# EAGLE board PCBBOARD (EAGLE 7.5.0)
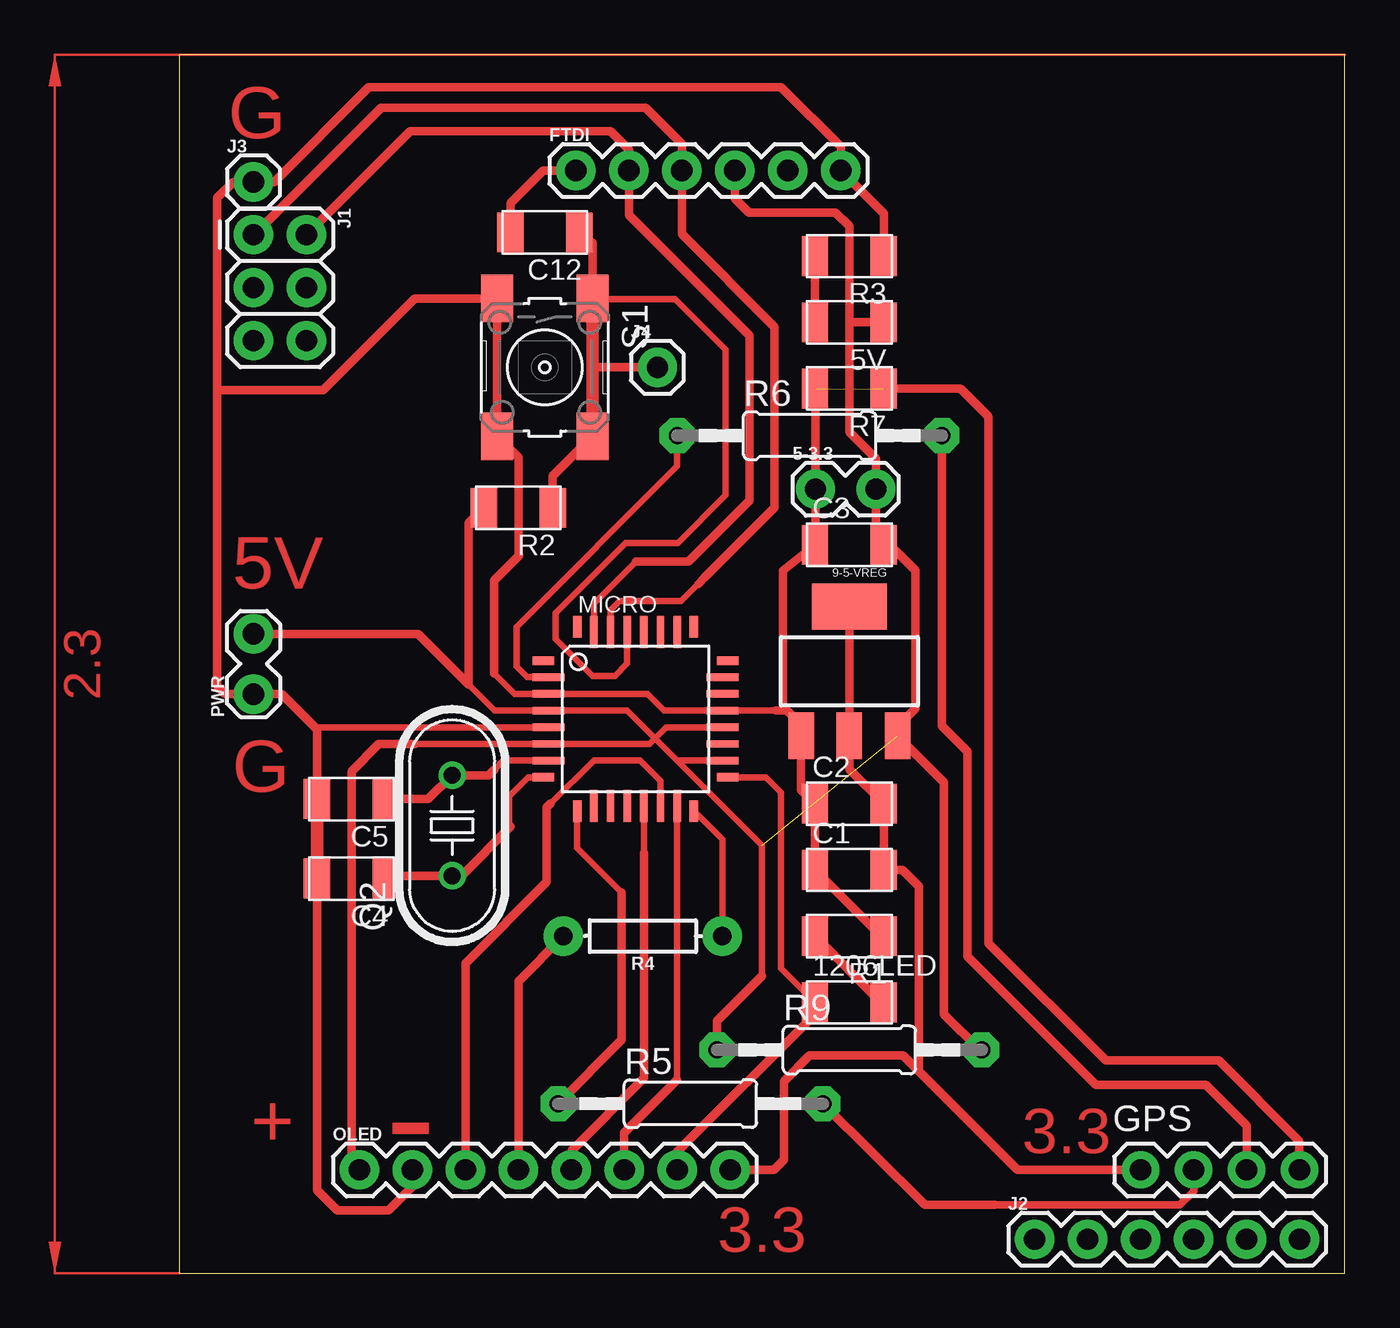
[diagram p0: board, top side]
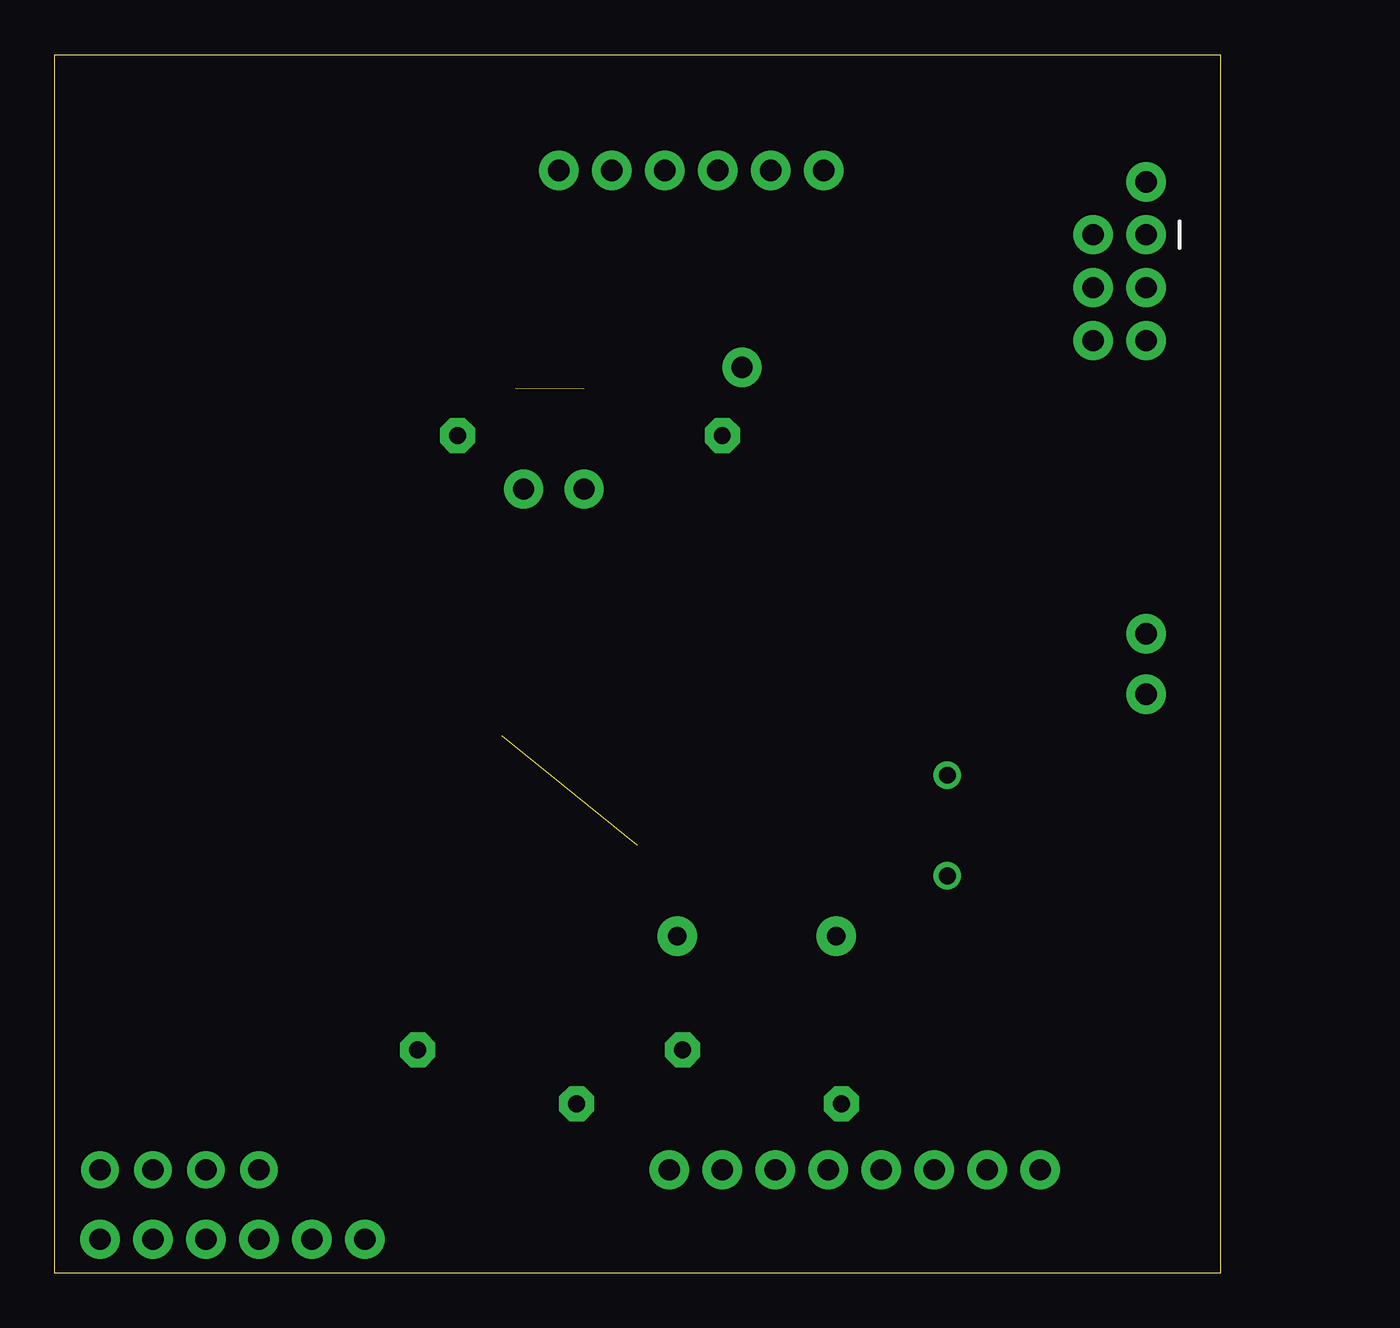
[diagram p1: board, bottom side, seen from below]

Size 55.88 x 58.42 mm. Coordinates in mm from the lower left corner, seen from the top.
Outline: 0,0 55.88,0 55.88,58.42 0,58.42 0,0
Copper layers (1*16): Top 0.035mm / dielectric 1.5mm / Bottom 0.035mm
Design rules "default": minimum track width 10mil, minimum drill 24mil, track to track 8mil, track to pad 8mil, pad to pad 8mil, via to via 8mil, smd to smd 8mil, copper to edge 40mil, drill to drill 8mil, minimum pad ring 10mil, minimum via ring 8mil, stop-mask expansion 4mil, vias tented up to drill 0mil, thermal gap 10mil

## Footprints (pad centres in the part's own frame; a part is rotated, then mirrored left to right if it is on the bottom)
1X02_LOCK = drill 1.016 pad 1.88: 1 -0.178,0; 2 2.718,0
LED1206FAB = smd 1.27 x 1.905: 1 -1.651,0; 2 1.651,0
SOT223 = smd 1.219 x 2.235: 1 -2.311,-3.099; 2 0,-3.099; 3 2.311,-3.099 | smd 3.6 x 2.2: 4 0,3.099
C1206FAB = smd 1.27 x 1.905: 1 -1.651,0; 2 1.651,0
1X06 = drill 1.016 pad 1.88: 1 0,0; 2 2.54,0; 3 5.08,0; 4 7.62,0; 5 10.16,0; 6 12.7,0
1X04-BIG = drill 1.016 pad 1.778: 1 0,0; 2 2.54,0; 3 5.08,0; 4 7.62,0
2X3 = drill 1.016 pad 1.88: 1 0,0; 2 0,2.54; 3 2.54,0; 4 2.54,2.54; 5 5.08,0; 6 5.08,2.54
1X01 = drill 1.016 pad 1.88: 1 0,0
TQFP32-08 = smd 1.016 x 0.406: 1 -4.42,2.8; 8 -4.42,-2.8; 17 4.42,-2.8; 24 4.42,2.8 | smd 1.524 x 0.356: 2 -4.166,2; 3 -4.166,1.2; 4 -4.166,0.4; 5 -4.166,-0.4; 6 -4.166,-1.2; 7 -4.166,-2; 18 4.166,-2; 19 4.166,-1.2; 20 4.166,-0.4; 21 4.166,0.4; 22 4.166,1.2; 23 4.166,2 | smd 0.406 x 1.016: 9 -2.8,-4.42; 16 2.8,-4.42; 25 2.8,4.42; 32 -2.8,4.42 | smd 0.356 x 1.524: 10 -2,-4.166; 11 -1.2,-4.166; 12 -0.4,-4.166; 13 0.4,-4.166; 14 1.2,-4.166; 15 2,-4.166; 26 2,4.166; 27 1.2,4.166; 28 0.4,4.166; 29 -0.4,4.166; 30 -1.2,4.166; 31 -2,4.166
1X08 = drill 1.016 pad 1.88: 1 0,0; 2 2.54,0; 3 5.08,0; 4 7.62,0; 5 10.16,0; 6 12.7,0; 7 15.24,0; 8 17.78,0
HC49U70 = drill 0.813: 1 -2.413,0; 2 2.413,0
R1206FAB = smd 1.27 x 1.905: 1 -1.651,0; 2 1.651,0
AXIAL-0.3 = drill 0.9 pad 1.88: P$1 -3.81,0; P$2 3.81,0
0207/12 = drill 0.813 pad 1.676 octagon: 1 -6.35,0; 2 6.35,0
6MM_SWITCH = smd 2.286 x 1.524: 1 -3.302,2.286; 2 3.302,2.286; 3 -3.302,-2.286; 4 3.302,-2.286

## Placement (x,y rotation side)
5-3.3  [1X02_LOCK]  30.68,37.59 0 top
5V  PWR LED  [LED1206FAB]  32.13,45.59 180 top
9-5-VREG  [SOT223]  32.13,28.86 0 top
1206LED  D13 LED  [LED1206FAB]  32.13,12.99 0 top
C1  10uF  [C1206FAB]  32.13,19.34 0 top
C2  10uF  [C1206FAB]  32.13,22.51 0 top
C3  10uF  [C1206FAB]  32.13,34.92 0 top
C4  22pF  [C1206FAB]  8.26,18.92 180 top
C5  22pF  [C1206FAB]  8.26,22.73 180 top
C12  0.1uF  [C1206FAB]  17.53,49.91 180 top
FTDI  [1X06]  19.02,52.87 0 top
GPS  1X4-BIG  [1X04-BIG]  46.1,4.95 0 top
J1  FEMALE 2x3  [2X3]  3.56,49.79 270 top
J2  [1X06]  41.02,1.62 0 top
J3  [1X01]  3.56,52.32 0 top
J4  [1X01]  22.92,43.43 0 top
MICRO  ATMEGA328P-AU  [TQFP32-08]  21.88,26.57 0 top
OLED  [1X08]  8.64,4.95 0 top
PWR  [1X02_LOCK]  3.56,27.94 90 top
Q2  [HC49U70]  13.08,21.46 90 top
R1  499  [R1206FAB]  32.13,16.16 180 top
R2  10K  [R1206FAB]  16.26,36.7 180 top
R3  499  [R1206FAB]  32.13,48.77 180 top
R4  0  [AXIAL-0.3]  22.23,16.16 180 top
R5  0  [0207/12]  24.51,8.13 0 top
R6  0  [0207/12]  30.23,40.16 0 top
R7  0  [R1206FAB]  32.13,42.42 180 top
R9  0  [0207/12]  32.13,10.71 0 top
S1  [6MM_SWITCH]  17.53,43.43 270 top

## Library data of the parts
5-3.3 FTDI J3 J4 PWR = SparkFun-Connectors
5V 1206LED C1-C5 C12 R1-R3 R7 S1 = fab
9-5-VREG = fab; PROD_ID: VREG-08170
GPS R5 R6 R9 = adafruit
J1 = SparkFun-Connectors; PROD_ID: CONN-11566
J2 = SparkFun-Connectors; PROD_ID: CONN-08437
MICRO = atmega8
OLED = SparkFun-Connectors; PROD_ID: CONN-08438
Q2 = crystal; OC_FARNELL: unknown; OC_NEWARK: unknown
R4 = SparkFun-Resistors; PROD_ID: RES-09327

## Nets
0(RX): FTDI.3 J1.1 MICRO.30
1(TX): FTDI.2 J1.2 MICRO.31
3.3V: 9-5-VREG.2 9-5-VREG.4 C1.2 C2.2 GPS.1 OLED.8
5V: 5-3.3.2 5V.1 9-5-VREG.3 C3.2 FTDI.4 MICRO.4 MICRO.6 MICRO.18 MICRO.20 OLED.1 PWR.2 R2.2 R9.1 R9.2
A0: MICRO.23
A1: MICRO.24
A2: MICRO.25
A3: MICRO.26
A4: MICRO.27
A5: MICRO.28
A6: MICRO.19
A7: MICRO.22
D2: MICRO.32
D3: MICRO.1
D4: GPS.3 R6.2
D5: GPS.2 R5.2
D6: MICRO.10
D7: MICRO.11
D8: MICRO.12
D9: MICRO.13 OLED.5
D10: MICRO.14 OLED.3
D11: MICRO.15 OLED.6
D12: OLED.4 R4.P$2
D13: 1206LED.1 MICRO.17 OLED.7
GND: 5-3.3.1 9-5-VREG.1 C1.1 C2.1 C3.1 C4.2 C5.2 FTDI.6 GPS.4 J3.1 MICRO.3 MICRO.5 MICRO.21 OLED.2 PWR.1 R1.1 R3.1 R7.1 R7.2 S1.3 S1.4
N$1: 1206LED.2 R1.2
N$2: 5V.2 R3.2
N$3: C5.1 MICRO.7 Q2.2
N$4: C4.1 MICRO.8 Q2.1
N$6: MICRO.16 R4.P$1
N$7: MICRO.9 R5.1
N$8: MICRO.2 R6.1
N$16: C12.2 FTDI.1
RST: C12.1 J4.1 MICRO.29 R2.1 S1.1 S1.2

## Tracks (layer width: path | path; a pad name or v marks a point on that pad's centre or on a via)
0(RX)
  Top 0.305: MICRO.30 20.68,31.79 21.11,32.23 24.07,32.23 25.19,33.35
  Top 0.406: J1.1 3.6,49.79 9.68,55.88 22.35,55.88 24.1,54.14 FTDI.3 24.1,49.82 28.54,45.37 28.54,36.7 25.19,33.35 24.89,33.05
1(TX)
  Top 0.305: MICRO.31 19.88,32.1 21.91,34.13
  Top 0.406: J1.2 11.07,54.77 20.67,54.77 21.56,53.88 FTDI.2 21.56,50.74 27.34,44.96 27.34,37.05 24.42,34.13 21.91,34.13
3.3V
  Top 0.406: 9-5-VREG.4 9-5-VREG.2 32.13,24.16 C2.2 C1.2 34.67,19.34 35.47,18.54 35.47,9.68 | GPS.1 40.2,4.95 35.47,9.68 | 35.47,9.68 34.7,10.45 30.23,10.45 28.99,9.21 28.99,5.43 28.51,4.95 OLED.8
5V  (1 unrouted)
  Top 0.305: 11.3,25.37 11.31,25.38 MICRO.6 22.55,25.38 22.81,25.64 | 13.88,28.23 15.13,26.98 MICRO.4 21.48,26.98 22.81,25.64 | 22.81,25.64 23.88,24.57 | 23.88,24.57 27.94,20.51 27.94,14.26 | MICRO.20 23.35,26.18 22.81,25.64 | MICRO.18 23.88,24.57
  Top 0.406: 11.3,25.37 9.56,25.37 8.26,24.07 8.26,5.33 OLED.1 | 32.13,45.59 32.13,50.2 31.46,50.86 27.3,50.86 26.64,51.53 FTDI.4 | 32.13,45.59 32.13,40.32 33.4,39.05 5-3.3.2 33.4,35.31 C3.2 34.07,34.92 35.31,33.69 35.31,27.08 34.44,26.22 9-5-VREG.3 36.67,23.53 36.67,12.41 38.38,10.71 R9.2 | 5V.1 32.13,45.59 | R2.2 13.88,35.97 13.88,28.23 11.44,30.66 PWR.2 | R9.1 25.78,12.1 27.94,14.26
D4
  Top 0.406: R6.2 36.58,26.23 37.78,25.02 37.78,15.18 43.94,9.02 49.21,9.02 51.18,7.05 GPS.3
D5
  Top 0.356: GPS.2 48.64,3.93 47.97,3.27 39.12,3.27
  Top 0.406: 39.12,3.27 35.75,3.27 R5.2
D9
  Top 0.305: MICRO.13 22.28,20.15
  Top 0.406: 22.28,20.15 22.28,9.35 18.8,5.87 OLED.5
D10
  Top 0.305: MICRO.14 23.08,23.6 22.1,24.57 19.88,24.57 17.81,22.51
  Top 0.406: OLED.3 13.72,14.86 17.62,18.76 17.62,22.32 17.81,22.51
D11
  Top 0.305: MICRO.15 23.88,9.27
  Top 0.406: 23.88,9.27 21.34,6.73 OLED.6
D12
  Top 0.406: OLED.4 16.26,14 R4.P$2
D13
  Top 0.305: MICRO.17 28.14,23.77 28.86,23.05 28.86,14.61 1206LED.1
  Top 0.406: OLED.7 23.88,5.81 30.48,12.41 1206LED.1
GND  (1 unrouted)
  Top 0.305: 28.61,26.98 MICRO.21 23.25,26.98 22.45,27.77 MICRO.3 16.07,27.77 15.08,28.77 | MICRO.5 6.71,26.18 6.6,26.07
  Top 0.406: R1.1 33.66,16.16 C1.1 C2.1 29.82,23.17 9-5-VREG.1 29.82,26.28 29.13,26.98 | 29.13,26.98 28.96,27.15 28.96,33.69 C3.1 30.68,35.41 30.5,35.59 5-3.3.1 30.5,42.39 R7.2 | 28.61,26.98 29.13,26.98 | OLED.2 11.18,4.16 10.03,3.02 7.56,3.02 6.6,3.97 C4.2 | C5.2 6.6,26.07 4.91,27.76 PWR.1 2.21,27.76 1.81,28.16 1.81,42.39 | 15.08,28.77 15.08,33.21 16.29,34.42 16.29,34.48 16.26,34.51 16.26,39.12 S1.4 S1.3 11.27,46.74 6.89,42.35 1.84,42.35 1.81,42.39 | R3.1 33.78,50.81 FTDI.6 31.72,54.01 28.86,56.86 9.08,56.86 4.54,52.32 J3.1 2.57,52.32 1.81,51.56 1.81,42.39 | R7.1 37.47,42.42 38.8,41.08 38.8,15.81 44.42,10.19 49.85,10.19 53.72,6.32 GPS.4
  Top 0.61: C4.2 C5.2
N$1
  Top 0.406: 1206LED.2 33.66,12.99 R1.2
N$2
  Top 0.406: R3.2 5V.2
N$3
  Top 0.305: 15.11,24.16 15.53,24.57 MICRO.7
  Top 0.406: C5.1 11.94,22.73 Q2.2 14.83,23.88 15.11,24.16
N$4
  Top 0.305: MICRO.8 16.73,23.77 15.81,22.86 15.81,21.5 15.89,21.41
  Top 0.406: 15.89,21.41 13.53,19.05 Q2.1 10.41,19.05 C4.1
N$6
  Top 0.305: R4.P$1 26.04,20.8 MICRO.16
N$7
  Top 0.305: MICRO.9 19.08,20.39 21.21,18.26
  Top 0.406: 21.21,18.26 21.21,11.18 R5.1
N$8
  Top 0.305: MICRO.2 16.67,28.57 16.16,29.08 16.16,30.99 23.88,38.7 R6.1
N$16
  Top 0.406: FTDI.1 17.44,52.87 15.88,51.31 C12.2
RST
  Top 0.305: MICRO.29 21.48,29.22 20.89,28.64 19.81,28.64 18.03,30.42 18.03,31.66 21.4,35.02 23.91,35.02 26.19,37.31 26.19,44.29 23.78,46.7 19.84,46.7 S1.1
  Top 0.406: S1.1 19.81,49.4 C12.1 | R2.1 17.91,38.23 S1.2 | J4.1 19.81,43.43
  Top 0.61: S1.1 19.81,43.43 S1.2
(copper drawn outside any net)
  shapes: Top area x2

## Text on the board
Top: G | 5V | G | + | 3.3 | - | 3.3

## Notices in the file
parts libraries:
SparkFun-Connectors: Licensing: Creative Commons ShareAlike 4.0 International - https://creativecommons.org/licenses/by-sa/4.0
